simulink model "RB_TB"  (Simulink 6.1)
settings: Solver=ode3  SolverMode=SingleTasking  StartTime=0  StopTime=0.1  FixedStep=0.01  RelTol=1e-3
libraries: simulink x2
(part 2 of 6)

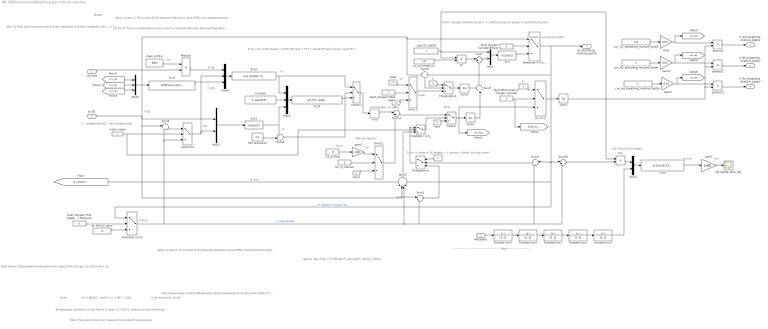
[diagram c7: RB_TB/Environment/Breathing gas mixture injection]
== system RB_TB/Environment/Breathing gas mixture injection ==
  note: Model:
  note: Valve_mode=1; The model of O2 pressure reduction valve (PRV) not compensated to ambient pressure (Drager Dolphin circuit).
  note: K
  note: Flow = Fs, when Pamb < 0.5*P_IM Flow = Fs*(1 -exp(9.5*log(k(i))))/(1 -exp(9.5*log(0.5))) Flow = 0 when P_IM <= P_BL Flow = 0 when P_O2_bottle <= P_IM
  note: Flow
  note: Fs
  note: P_BL
  note: P_breathing_mixture_bottle
  note: Valve_mode=0; The model of O2 pressure reduction valve (PRV) compensated to ambient pressure (Ray circuit).
  note: P_IM_sl
  note: 1 - compensated 0 - not compensated
  note: Fault: "Oxygen Cylinder Empty" = 1 Bottle pressure equals to ambient pressure
  note: l/s
  note: Leaks
  note: Flow = 0 when P_O2_bottle < P_spring + Pamb (for Ray valve)
  note: approx. Ray Flow = Fs*(Pamb+P_spring)/(P_spring + Patm)
  note: pure oxygen, l/s
  note: um
  note: bar
  note: Temperature correction of the flow is (t_amb +273)/273, where t_amb is the temperature of the gas in balloon in deg. C
  note: Note: the system does not measure the ambient temperature
  note: Flow theory: http://www.therebreathersite.nl/gas_flow_through_an_orifice.htm Sonic flow D = d^2*po*A, where d is orifice diameter in mm; p0 = intermediate pressure (input orifice pressure), in bar; A is constant. A = A_O2*cnc_O2+ A_N2*cnc_N2+A_He*cnc_He, where A_O2 = 8.65, A_N2=9.233, A_He=20.71 are constants; cnc_O2, cnc_N2 and cnc_He is concentration of O2, N2 and He ( N2/O2 : He/O2 == 1.067 2.394)
  note: Max O2 flow must be more than the set metabolic rate Max metabolic rate = 0.1 /ls
  note: P_IM
  note: l/s
  note: Life Time of O2 bottele
  note: second
  note: min
  note: ------------------------------------------------- filter------------------------------------------------
  note: Manual injector
  note: l/min
  note: 21_02_07 The uncompensated valve means a Constant Absolute Pressure Regulator. The compensated one is a Constant Ambient Pressure Regulator.
  note: http://www.ckgas.com/html/Rotameters-Basic-Flowmeter-Principles.html Table of Flow Rate Factors For Gases Other Than Air: Gas Factor Air 1 Carbob Dioxide 1.23 Helium 0.37 Nitrogen 0.98 Oxygen 1.05 (N2/O2 : He/O2 == 1. 071 : 2.838) (N2/Air : He/Air == 1. 020 : 2.703)
  note: for ( N2/O2 : He/O2 == 1.067 : 2.83)
  note: A_He should be 24.48
  note: Note:
  note: A_gas
  Orf_size : Inport  Port=1  LatchInput=off
  pr_BL : Inport  Port=2  LatchInput=off
  Metabolic : Inport  Port=3  LatchInput=off
  >=0 : DeadZone  LowerValue=-inf  UpperValue=0
  Fcn : Fcn  Expr=u(2)/u(1)
  Fcn1 : Fcn  Expr=u(1)/u(2)
  Fcn2 : Fcn  Expr=(u(1)/1000)^2*u(2)*u(3)/60
  Fcn3 : Fcn  Expr=8.65*u(1)+9.33*u(2)+24.48*u(3)
  Fcn4 : Fcn  Expr=u(1)/(u(2)+0.0000001)-300
  Fcn5 : Fcn  Expr=u(1)*(1 -exp(9.5*log(u(3))))/u(2)
  Gain : Gain  Gain=0.01
  Gain1 : Gain  Gain=0.01
  Gain2 : Gain  Gain=0.01
  Leak : Constant  Value=2.5
  Mux : Mux  Inputs=2
  Mux1 : Mux  Inputs=2
  Mux2 : Mux  Inputs=3
  Mux3 : Mux  Inputs=2
  Mux4 : Mux  Inputs=3
  Mux5 : Mux  Inputs=3
  O2_bottle_time_life : Scope
  O2_in_flow : Constant  Value=75
  O2_in_manual : Constant  Value=0
  Pr : Product
  Pr1 : Product
  Product : Product
  Sum : Sum  Inputs=|+-
  Sum1 : Sum  Inputs=|-+
  Sum10 : Sum  Inputs=|+-
  Sum11 : Sum  Inputs=|++
  Sum2 : Sum  Orientation=left  Inputs=|-+
  Sum3 : Sum  Inputs=|++
  Sum4 : Sum  Inputs=-+|
  Sum5 : Sum  Orientation=up  Inputs=+--+
  Sum7 : Sum  Orientation=up  Inputs=++|
  Sum8 : Sum  Orientation=down  Inputs=+-
  Switch : Switch  Criteria=u2 > Threshold
  Switch3 : Switch  Criteria=u2 > Threshold
  Threshold=0 : Switch  Orientation=left  Criteria=u2 > Threshold
  Threshold=0_ : Switch  Criteria=u2 > Threshold
  Transfer Fcn{1..5} (5 alike) : TransferFcn  Denominator=[1 1]
  cnc_He_breathing_mixture_bottle : Constant  Value=0
  cnc_N2_breathing_mixture_bottle : Constant  Value=0
  cnc_O2_breathing_mixture_bottle : Constant  Value=100
  constant : Constant  Value=1 -exp(9.5*log(0.5))
  diam_orifice : Constant  Value=400
  fault_Oxygen Cylinder Empty : Constant  Value=0
  fault_Oxygen First Stage Over Pressure : Constant  Value=0
  fault_Oxygen Hose Leaks : Constant  Value=0
  fault_Wrong Gas in Oxygen cylinder : Constant  Value=0
  gain1 : Gain  Gain=1/60
  gain2 : Gain  Gain=1/60
  half pressure1 : Constant  Value=0.5
  pr_IM_O2_valve : Constant  Value=10
  pr_O2_bottle_ini : Constant  Value=230
  product : Product
  product1 : Product
  product2 : Product
  size_O2_bottle : Constant  Value=3
  sum1 : Integrator
  sum2 : Integrator
  sum3 : Integrator
  th = 0.5 : Switch  Criteria=u2 > Threshold  Threshold=0.5
  th=0.5 : Switch  Criteria=u2 > Threshold  Threshold=0.5
  th=0.5_ : Switch  Criteria=u2 > Threshold  Threshold=0.5
  threshold = 0.5 : Switch  Criteria=u2 > Threshold  Threshold=0.5
  threshold = 0.5_ : Switch  Criteria=u2 > Threshold
  threshold = 0.5__ : Switch  Criteria=u2 > Threshold  Threshold=0.5
  tresh=0.5 : Switch  Criteria=u2 > Threshold  Threshold=0.5
  valve_mode : Constant
  z : Constant  Value=0
  z_ : Constant  Value=0
  zero : Constant  Value=0
  zero1 : Constant  Value=0
  zero_ : Constant  Value=0
  zero__ : Constant  Orientation=left  Value=0
  pr_breathing_mixture_bottle : Outport
  V_O2_breathing_mixture_bottle : Outport  Port=2
  V_N2_breathing_mixture_bottle : Outport  Port=3
  V_He_breathing_mixture_bottle : Outport  Port=4
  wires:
  Sum/1 -> Mux/2
  size_O2_bottle/1 -> Mux/1, Pr/1, Pr1/1
  Mux/1 -> Fcn/1
  Pr/1 -> Sum/1
  pr_O2_bottle_ini/1 -> Pr/2
  sum1/1 -> Sum7/2
  pr_BL/1 -> Mux1/1, threshold = 0.5__/1, Sum8/1, Sum5/2, Sum1/1, Sum3/1
  zero/1 -> Switch/3
  Switch3/1 -> >=0/1
  threshold = 0.5/1 -> Sum5/3, Sum1/2, Sum2/2, Sum10/2, Sum3/2, tresh=0.5/3  "pr_intermediate"
  [pr_ambient_sea_level] -> Sum5/1  "pr_atm"
  half pressure1/1 -> Sum4/2
  Mux1/1 -> Fcn1/1
  Mux2/1 -> Fcn5/1
  Sum4/1 -> Switch3/2
  constant/1 -> Mux2/2
  Fcn5/1 -> Switch3/3
  threshold = 0.5__/1 -> Sum8/2, Sum2/1, threshold = 0.5/1, Sum5/4, Sum10/1, pr_breathing_mixture_bottle/1  "pr_breathing_mixture_bottle"
  Fcn/1 -> threshold = 0.5__/3
  fault_Oxygen Cylinder Empty/1 -> threshold = 0.5__/2
  Sum2/1 -> Threshold=0/2
  zero__/1 -> Threshold=0/1
  threshold = 0.5_/1 -> Switch/2
  Sum1/1 -> Threshold=0/3
  Threshold=0/1 -> threshold = 0.5_/1
  Sum5/1 -> threshold = 0.5_/3
  fault_Oxygen First Stage Over Pressure/1 -> threshold = 0.5/2
  fault_Oxygen Hose Leaks/1 -> th=0.5/2
  zero_/1 -> th=0.5/3
  Leak/1 -> th=0.5/1
  Sum7/1 -> Sum/2
  >=0/1 -> Sum11/1
  Sum8/1 -> Threshold=0_/2
  z/1 -> Threshold=0_/1
  th=0.5/1 -> Threshold=0_/3
  sum2/1 -> Sum7/1
  Threshold=0_/1 -> sum2/1
  fault_Wrong Gas in Oxygen cylinder/1 -> th = 0.5/2, [Fault_O2_wrong]
  z_/1 -> th = 0.5/1
  th = 0.5/1 -> sum3/1
  sum3/1 -> product2/2, product1/2, product/2
  Mux4/1 -> Fcn2/1
  valve_mode/1 -> tresh=0.5/2, threshold = 0.5_/2
  Fcn1/1 -> Sum4/1, Mux2/3
  Fcn2/1 -> Mux2/1, Switch3/1
  Product/1 -> Mux4/1
  diam_orifice/1 -> Product/1
  pr_IM_O2_valve/1 -> threshold = 0.5/3
  O2_in_manual/1 -> th=0.5_/2
  zero1/1 -> th=0.5_/3
  Switch/1 -> sum1/1, th = 0.5/3, [O2_flow]
  th=0.5_/1 -> Sum11/2
  Mux3/1 -> Fcn4/1
  Pr1/1 -> Mux3/1
  Metabolic/1 -> Transfer Fcn5/1
  Transfer Fcn2/1 -> Transfer Fcn1/1
  Transfer Fcn1/1 -> Transfer Fcn3/1
  Transfer Fcn5/1 -> Transfer Fcn4/1
  Transfer Fcn4/1 -> Transfer Fcn2/1
  Fcn4/1 -> gain1/1
  gain1/1 -> O2_bottle_time_life/1
  Sum10/1 -> Pr1/2
  Transfer Fcn3/1 -> Mux3/2
  gain2/1 -> th=0.5_/1
  O2_in_flow/1 -> gain2/1
  Sum11/1 -> Switch/1
  Orf_size/1 -> Product/2
  tresh=0.5/1 -> Mux4/2, Mux1/2
  Sum3/1 -> tresh=0.5/1
  Fcn3/1 -> Mux4/3
  Mux5/1 -> Fcn3/1
  cnc_O2_breathing_mixture_bottle/1 -> Gain/1
  Gain/1 -> product/1, [cnc_O2]
  product/1 -> V_O2_breathing_mixture_bottle/1
  cnc_N2_breathing_mixture_bottle/1 -> Gain1/1
  Gain1/1 -> product1/1, [cnc_N2]
  product1/1 -> V_N2_breathing_mixture_bottle/1
  product2/1 -> V_He_breathing_mixture_bottle/1
  cnc_He_breathing_mixture_bottle/1 -> Gain2/1
  Gain2/1 -> product2/1, [cnc_He]
  [cnc_O2] -> Mux5/1
  [cnc_He] -> Mux5/3
  [cnc_N2] -> Mux5/2

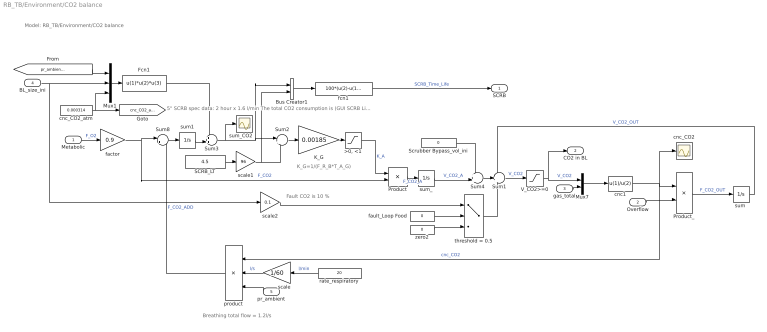
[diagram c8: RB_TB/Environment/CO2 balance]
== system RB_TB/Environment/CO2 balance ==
  note: Model: RB_TB/Environment/CO2 balance
  note: K_G=1/(F_R_B*T_A_G)
  note: Breathing total flow = 1.2l/s
  note: 5" SCRB spec data: 2 hour x 1.6 l/min The total CO2 consumption is (GUI SCRB Life-Time) x 192 / 2 litre
  note: Fault CO2 is 10 %
  Metabolic : Inport  Port=1  LatchInput=off
  Overflow : Inport  Port=2  LatchInput=off
  gas_total : Inport  Port=3  LatchInput=off
  BL_size_ini : Inport  Port=4  LatchInput=off
  pr_ambient : Inport  Orientation=left  Port=5  LatchInput=off
  ">0, <1" : Saturate  UpperLimit=1  LowerLimit=0
  Bus Creator1 : BusCreator  DialogController=Simulink.DDGSource_Bus  Inputs=2
  Fcn1 : Fcn  Expr=u(1)*u(2)*u(3)
  K_G : Gain  Gain=0.00185
  Mux1 : Mux  Inputs=3
  Mux7 : Mux  Inputs=2
  Product : Product
  Product_ : Product
  SCRB_LT : Constant  Value=4.5
  Scrubber Bypass_vol_ini : Constant  Value=0
  Sum1 : Sum  Inputs=-++
  Sum2 : Sum  Inputs=|+-
  Sum3 : Sum  Inputs=++|
  Sum4 : Sum  Inputs=++|
  Sum8 : Sum  Inputs=|++
  V_CO2>=0 : Saturate  UpperLimit=inf  LowerLimit=0
  cnc1 : Fcn  Tag=ee  Priority=306454640  Expr=u(1)/u(2)
  cnc_CO2 : Scope
  cnc_CO2_atm : Constant  Value=0.000314
  factor : Gain  Gain=0.9
  fault_Loop Food : Constant  Value=0
  fcn1 : Fcn  Expr=100*(u(2)-u(1))/u(2)
  product : Product  Orientation=left  Inputs=3
  rate_respiratory : Constant  Orientation=left  Value=20
  scale : Gain  Orientation=left  Gain=1/60
  scale1 : Gain  Gain=96
  scale2 : Gain  Gain=0.1
  "sum " : Integrator
  sum1 : Integrator
  sum_ : Integrator
  sum_CO2 : Scope
  threshold = 0.5 : Switch  Criteria=u2 > Threshold  Threshold=0.5
  zero2 : Constant  Value=0
  SCRB : Outport
  CO2 in BL : Outport  Port=2
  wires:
  Sum2/1 -> K_G/1
  K_G/1 -> ">0, <1"/1
  ">0, <1"/1 -> Product/1  "K_A"
  Product/1 -> sum_/1  "F_CO2_A"
  Sum1/1 -> V_CO2>=0/1  "V_CO2"
  Product_/1 -> "sum "/1  "F_CO2_OUT"
  "sum "/1 -> Sum1/1  "V_CO2_OUT"
  V_CO2>=0/1 -> Mux7/1, CO2 in BL/1  "V_CO2"
  Sum8/1 -> sum1/1
  Sum3/1 -> Sum2/1, Bus Creator1/1, sum_CO2/1
  rate_respiratory/1 -> scale/1  "l/min"
  scale/1 -> product/2  "l/s"
  cnc_CO2_atm/1 -> [cnc_CO2_atm], Mux1/3
  BL_size_ini/1 -> scale2/1, Mux1/2
  SCRB_LT/1 -> scale1/1
  Bus Creator1/1 -> fcn1/1
  fcn1/1 -> SCRB/1  "SCRB_Time_Life"
  scale1/1 -> Sum2/2, Bus Creator1/2
  threshold = 0.5/1 -> Sum1/3
  fault_Loop Food/1 -> threshold = 0.5/2
  scale2/1 -> threshold = 0.5/1
  zero2/1 -> threshold = 0.5/3
  Mux7/1 -> cnc1/1
  cnc1/1 -> cnc_CO2/1, Product_/1, product/1  "cnc_CO2"
  Overflow/1 -> Product_/2
  gas_total/1 -> Mux7/2
  [pr_ambient_sea_level] -> Mux1/1
  Mux1/1 -> Fcn1/1
  product/1 -> Sum8/2  "F_CO2_ADD"
  sum1/1 -> Sum3/2
  Fcn1/1 -> Sum3/1
  Sum4/1 -> Sum1/2
  sum_/1 -> Sum4/2  "V_CO2_A"
  Scrubber Bypass_vol_ini/1 -> Sum4/1
  pr_ambient/1 -> product/3
  factor/1 -> Sum8/1, Product/2  "F_CO2"
  Metabolic/1 -> factor/1  "F_O2"

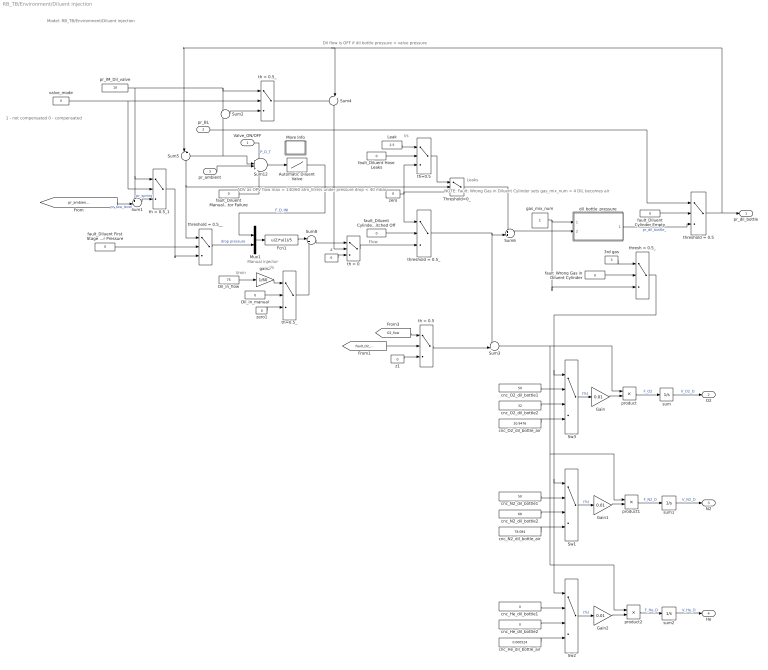
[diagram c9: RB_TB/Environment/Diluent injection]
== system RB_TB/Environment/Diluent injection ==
  note: Model: RB_TB/Environment/Diluent injection
  note: NOTE: Fault: Wrong Gas in Diluent Cylinder sets gas_mix_num = 4 DIL becomes air
  note: Dil flow is OFF if dil bottle pressure < valve pressure
  note: 1 - not compensated 0 - compensated
  note: l/s
  note: Leaks
  note: Flow
  note: l/s
  note: Manual injector
  note: l/min
  note: ADV as OPV flow max = 140/60 atm_litre/s under pressure drop < 40 mbar
  Valve_ON/OFF : Inport  Port=1  LatchInput=off
  pr_BL : Inport  Port=2  LatchInput=off
  pr_ambient : Inport  Port=3  LatchInput=off
  3rd gas : Constant  Value=3
  Automatic Diluent Valve : Lookup  DialogController=Simulink.DDGSource  InputValues=[-1000 0.039 0.04 0.3 1000]  OutputValues=[0 0 70 140 140]/60  LookUpMeth=Interpolation-Use End Values
  Dil_in_flow : Constant  Value=75
  Dil_in_manual : Constant  Value=0
  Fcn1 : Fcn  Expr=u(2)*u(1)/5
  Gain : Gain  Gain=0.01
  Gain1 : Gain  Gain=0.01
  Gain2 : Gain  Gain=0.01
  Leak : Constant  Value=2.5
  More Info : Subsystem
  Mux1 : Mux  Inputs=2
  Sum1 : Sum  Inputs=+-|
  Sum12 : Sum  Inputs=+-++
  Sum2 : Sum
  Sum3 : Sum  Inputs=++|
  Sum4 : Sum  Orientation=down  Inputs=-+|
  Sum5 : Sum  Orientation=down  Inputs=|+-
  Sum6 : Sum  Inputs=++|
  Sum8 : Sum  Inputs=|++
  Sw1 : MultiPortSwitch  Inputs=3
  Sw2 : MultiPortSwitch  Inputs=3
  Sw3 : MultiPortSwitch  Inputs=3
  Threshold=0_ : Switch  Criteria=u2 > Threshold
  cnc_He_dil_bottle1 : Constant  Value=0
  cnc_He_dil_bottle2 : Constant  Value=0
  cnc_He_dil_bottle_air : Constant  Value=0.000524
  cnc_N2_dil_bottle1 : Constant  Value=50
  cnc_N2_dil_bottle2 : Constant  Value=68
  cnc_N2_dil_bottle_air : Constant  Value=78.084
  cnc_O2_dil_bottle1 : Constant  Value=50
  cnc_O2_dil_bottle2 : Constant  Value=32
  cnc_O2_dil_bottle_air : Constant  Value=20.9476
  dil_bottle_pressure : Subsystem
  fault_Diluent Cylinder Empty : Constant  Value=0
  fault_Diluent Cylinder Switched Off : Constant  Value=0
  fault_Diluent First Stage Over Pressure : Constant  Value=0
  fault_Diluent Hose Leaks : Constant  Value=0
  fault_Diluent Manual Injector Failure : Constant  Value=0
  fault_Wrong Gas in Diluent Cylinder : Constant  Value=0
  gain2 : Gain  Gain=1/60
  gas_mix_num : Constant
  pr_IM_Dil_valve : Constant  Value=10
  product : Product
  product1 : Product
  product2 : Product
  sum : Integrator
  sum1 : Integrator
  sum2 : Integrator
  th = 0 : Switch  Criteria=u2 > Threshold
  th = 0.5 : Switch  Criteria=u2 > Threshold  Threshold=0.5
  th = 0.5_ : Switch  Criteria=u2 > Threshold
  th = 0.5_1 : Switch  Criteria=u2 > Threshold
  th=0.5 : Switch  Criteria=u2 > Threshold  Threshold=0.5
  th=0.5_ : Switch  Criteria=u2 > Threshold  Threshold=0.5
  thresh = 0.5_ : Switch  Criteria=u2 > Threshold  Threshold=0.5
  threshold = 0.5 : Switch  Criteria=u2 > Threshold  Threshold=0.5
  threshold = 0.5_ : Switch  Criteria=u2 > Threshold  Threshold=0.5
  threshold = 0.5__ : Switch  Criteria=u2 > Threshold  Threshold=0.5
  valve_mode : Constant  Value=0
  z : Constant  Value=0
  z1 : Constant  Value=0
  zero : Constant  Value=0
  zero1 : Constant  Value=0
  pr_dil_bottle : Outport
  O2 : Outport  Port=2
  N2 : Outport  Port=3
  He : Outport  Port=4
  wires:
  zero/1 -> Threshold=0_/3, th=0.5/3, threshold = 0.5_/1
  gas_mix_num/1 -> dil_bottle_pressure/1(gas_mix), thresh = 0.5_/3
  product/1 -> sum/1  "F_O2"
  sum/1 -> O2/1  "V_O2_D"
  sum1/1 -> N2/1  "V_N2_D"
  product1/1 -> sum1/1  "F_N2_D"
  sum2/1 -> He/1  "V_He_D"
  product2/1 -> sum2/1  "F_He_D"
  cnc_N2_dil_bottle2/1 -> Sw1/3
  cnc_O2_dil_bottle1/1 -> Sw3/2
  Sw3/1 -> Gain/1  "(%)"
  Gain/1 -> product/2
  Gain1/1 -> product1/2
  Gain2/1 -> product2/2
  Sw2/1 -> Gain2/1  "(%)"
  dil_bottle_pressure/1(O2) -> threshold = 0.5/3  "pr_dil_bottle_"
  cnc_O2_dil_bottle2/1 -> Sw3/3
  cnc_N2_dil_bottle1/1 -> Sw1/2
  cnc_He_dil_bottle1/1 -> Sw2/2
  cnc_He_dil_bottle2/1 -> Sw2/3
  threshold = 0.5/1 -> pr_dil_bottle/1, Sum5/1, Sum4/2
  fault_Diluent Cylinder Empty/1 -> threshold = 0.5/2
  z/1 -> th = 0/3
  pr_BL/1 -> Sum12/2, Sum5/2, threshold = 0.5/1, Sum2/2
  fault_Diluent Cylinder Switched Off/1 -> threshold = 0.5_/2
  threshold = 0.5_/1 -> Sum6/2, Sum3/1
  Sw1/1 -> Gain1/1  "(%)"
  cnc_O2_dil_bottle_air/1 -> Sw3/4
  cnc_N2_dil_bottle_air/1 -> Sw1/4
  cnc_He_dil_bottle_air/1 -> Sw2/4
  [O2_flow] -> th = 0.5/1
  [Fault_O2_wrong] -> th = 0.5/2
  z1/1 -> th = 0.5/3
  th = 0.5/1 -> Sum3/2
  Sum3/1 -> product1/1, product2/1, product/1
  valve_mode/1 -> th = 0.5_/2, th = 0.5_1/2
  Sum2/1 -> th = 0.5_/3
  Sum4/1 -> th = 0/2
  Mux1/1 -> Fcn1/1
  fault_Diluent First Stage Over Pressure/1 -> threshold = 0.5__/2
  threshold = 0.5__/1 -> Mux1/2  "drop pressure"
  Sum5/1 -> threshold = 0.5__/1, Threshold=0_/2
  fault_Diluent Hose Leaks/1 -> th=0.5/2
  Leak/1 -> th=0.5/1
  Sum6/1 -> dil_bottle_pressure/2(F_D)
  Threshold=0_/1 -> Sum6/1
  th=0.5/1 -> Threshold=0_/1
  pr_IM_Dil_valve/1 -> th = 0.5_/1, Sum2/1, th = 0.5_1/1, Sum1/1
  th = 0.5_/1 -> Sum4/1
  th = 0.5_1/1 -> threshold = 0.5__/3
  [pr_ambient_sea_level] -> Sum1/2  "pr_sea_level"
  Sum1/1 -> th = 0.5_1/3  "pr_spring"
  fault_Wrong Gas in Diluent Cylinder/1 -> thresh = 0.5_/2
  3rd gas/1 -> thresh = 0.5_/1
  thresh = 0.5_/1 -> Sw3/1, Sw1/1, Sw2/1
  pr_ambient/1 -> Sum12/3
  fault_Diluent Manual Injector Failure/1 -> Sum12/4
  Sum12/1 -> Automatic Diluent Valve/1
  Dil_in_manual/1 -> th=0.5_/2
  zero1/1 -> th=0.5_/3
  th=0.5_/1 -> Sum8/2
  gain2/1 -> th=0.5_/1
  Dil_in_flow/1 -> gain2/1
  Fcn1/1 -> Sum8/1
  Sum8/1 -> th = 0/1
  th = 0/1 -> threshold = 0.5_/3
  Automatic Diluent Valve/1 -> Mux1/1  "F_D_INI"
  Valve_ON/OFF/1 -> Sum12/1  "P_D_T"

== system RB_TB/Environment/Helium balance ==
  note: V_He_BL_ini
  note: Model: RB_TB/Environment/Helium balance
  V_He_breathing : Inport  Port=1  LatchInput=off
  V_He_dil : Inport  Port=2  LatchInput=off
  gas_total : Inport  Port=3  LatchInput=off
  Overflow : Inport  Port=4  LatchInput=off
  BL_size_ini : Inport  Port=5  LatchInput=off
  Fcn1 : Fcn  Expr=u(1)*u(2)*u(3)
  Mux1 : Mux  Inputs=3
  Mux3 : Mux  Inputs=2
  Product_ : Product
  Sum5 : Sum  Inputs=+++-
  V_He>=0 : Saturate  UpperLimit=inf  LowerLimit=0
  cnc3 : Fcn  Tag=ee  Priority=306454640  Expr=u(1)/u(2)
  cnc_He : Scope
  sum : Integrator
  He in BL : Outport
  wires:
  V_He_dil/1 -> Sum5/2  "V_He_D"
  Fcn1/1 -> Sum5/1
  V_He>=0/1 -> He in BL/1, Mux3/1  "V_He"
  Sum5/1 -> V_He>=0/1  "V_He"
  sum/1 -> Sum5/4  "V_He_OUT"
  Product_/1 -> sum/1  "F_He_OUT"
  Mux3/1 -> cnc3/1
  cnc3/1 -> cnc_He/1, Product_/1, [cnc_He_presize]
  gas_total/1 -> Mux3/2
  Overflow/1 -> Product_/2
  BL_size_ini/1 -> Mux1/2
  [pr_ambient_sea_level] -> Mux1/1
  Mux1/1 -> Fcn1/1
  [cnc_He_atm] -> Mux1/3
  V_He_breathing/1 -> Sum5/3

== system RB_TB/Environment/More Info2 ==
  note: Humidity: The water in breathing and from the chemical reaction maintain the humidity constantly at 100%. The situation in open circuit is different, the gas mixture is completely dry, and the diver loses a big quantity of liquids during the dive.

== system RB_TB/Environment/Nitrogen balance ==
  note: Model: RB_TB/Environment/Nitrogen balance
  V_N2_breathing : Inport  Port=1  LatchInput=off
  V_N2_dil : Inport  Port=2  LatchInput=off
  gas_total : Inport  Port=3  LatchInput=off
  Overflow : Inport  Port=4  LatchInput=off
  BL_size_ini : Inport  Port=5  LatchInput=off
  Display2 : Display
  Fcn1 : Fcn  Expr=u(1)*u(2)*u(3)
  Mux1 : Mux  Inputs=3
  Mux8 : Mux  Inputs=2
  Product_ : Product
  Sum5 : Sum  Inputs=+++-
  V_N2>=0 : Saturate  UpperLimit=inf  LowerLimit=0
  cnc2 : Fcn  Tag=ee  Priority=306454640  Expr=u(1)/u(2)
  cnc_N2 : Scope
  sum : Integrator
  N2 in BL : Outport
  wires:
  Product_/1 -> sum/1  "F_N2_OUT"
  sum/1 -> Display2/1, Sum5/4  "V_N2_OUT"
  Sum5/1 -> V_N2>=0/1  "V_N2"
  V_N2>=0/1 -> Mux8/1, N2 in BL/1  "V_N2"
  Fcn1/1 -> Sum5/1
  V_N2_dil/1 -> Sum5/2  "V_N2_D"
  Mux8/1 -> cnc2/1
  cnc2/1 -> Product_/1, cnc_N2/1, [cnc_N2_presize]
  gas_total/1 -> Mux8/2
  Overflow/1 -> Product_/2
  BL_size_ini/1 -> Mux1/2
  [pr_ambient_sea_level] -> Mux1/1
  Mux1/1 -> Fcn1/1
  [cnc_N2_atm] -> Mux1/3
  V_N2_breathing/1 -> Sum5/3

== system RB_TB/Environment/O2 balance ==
  note: Model: RB_TB/Environment/O2 balance
  V_O2_breathing : Inport  Port=1  LatchInput=off
  V_O2_dil : Inport  Port=2  LatchInput=off
  Metabolic : Inport  Port=3  LatchInput=off
  gas_total : Inport  Port=4  LatchInput=off
  Overflow : Inport  Port=5  LatchInput=off
  BL_size_ini : Inport  Port=6  LatchInput=off
  Fcn1 : Fcn  Expr=u(1)*u(2)*u(3)
  Mux1 : Mux  Inputs=3
  Mux6 : Mux  Inputs=2
  Product : Product
  Sum2 : Sum  Inputs=-+++-
  V_O2>=0 : Saturate  UpperLimit=inf  LowerLimit=0
  cnc : Fcn  Tag=ee  Priority=306454640  Expr=u(1)/u(2)
  cnc_O2 : Scope
  cnc_O2_atm : Constant  Value=0.20948
  sum : Integrator
  sum2 : Integrator
  O2 in BL : Outport
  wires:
  Fcn1/1 -> Sum2/3  "V_O2_ini"
  Product/1 -> sum/1  "F_O2_OUT"
  sum/1 -> Sum2/1  "V_O2_OUT"
  Sum2/1 -> V_O2>=0/1  "V_O2"
  V_O2_breathing/1 -> Sum2/2  "V_O2_O"
  sum2/1 -> Sum2/5  "V_R_B"
  V_O2_dil/1 -> Sum2/4  "V_O2_D"
  Metabolic/1 -> sum2/1  "F_R_B"
  V_O2>=0/1 -> Mux6/1, O2 in BL/1  "V_O2"
  BL_size_ini/1 -> Mux1/2
  cnc_O2_atm/1 -> [cnc_O2_atm], Mux1/3
  Mux6/1 -> cnc/1
  gas_total/1 -> Mux6/2
  cnc/1 -> Product/1, cnc_O2/1
  Overflow/1 -> Product/2
  [pr_ambient_sea_level] -> Mux1/1
  Mux1/1 -> Fcn1/1

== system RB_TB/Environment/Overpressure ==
  note: Model: RB_TB/Environment/Overpressure
  note: OPV flow max = 300/60 (atm_litre)/s under pressure drop < 40 mbar
  Depth : Inport  Port=1  LatchInput=off
  pr_BL : Inport  Port=2  LatchInput=off
  More Info2 : Subsystem
  OverPressure Valve : Lookup  DialogController=Simulink.DDGSource  InputValues=[-1000 0.025 0.04 0.3 1000]  OutputValues=[0 0 300 600 600]/60  LookUpMeth=Interpolation-Use End Values
  Sum12 : Sum  Inputs=|-+
  Sum4 : Sum  Inputs=++|
  x 0.2 : Gain  Gain=0.1
  Overflow : Outport
  pr_ambient : Outport  Port=2
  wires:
  Depth/1 -> x 0.2/1
  Sum4/1 -> Sum12/1, pr_ambient/1
  x 0.2/1 -> Sum4/2  "water pressure"
  Sum12/1 -> OverPressure Valve/1
  [pr_ambient_sea_level] -> Sum4/1  "bar"
  pr_BL/1 -> Sum12/2  "Breathing loop pressure"
  OverPressure Valve/1 -> Overflow/1

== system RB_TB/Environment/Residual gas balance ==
  note: Model: RB_TB/Environment/Residual gas balance gas balance
  note: vol_reminder_BL_ini
  gas_total : Inport  Port=1  LatchInput=off
  Overflow : Inport  Port=2  LatchInput=off
  BL_size_ini : Inport  Port=3  LatchInput=off
  Fcn1 : Fcn  Expr=u(1)*u(2)*u(3)
  Mux1 : Mux  Inputs=3
  Mux9 : Mux  Inputs=2
  Product_ : Product
  Sum5 : Sum  Inputs=|+-
  V_Re>=0 : Saturate  UpperLimit=inf  LowerLimit=0
  cnc4 : Fcn  Tag=ee  Priority=306454640  Expr=u(1)/u(2)
  cnc_res : Scope
  cnc_res_atm : Constant  Value=0.009365
  sum : Integrator
  Re in BL : Outport
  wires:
  sum/1 -> Sum5/2  "V_Re_OUT"
  Sum5/1 -> V_Re>=0/1  "V_Re"
  V_Re>=0/1 -> Re in BL/1, Mux9/1  "V_Re"
  Fcn1/1 -> Sum5/1
  cnc4/1 -> cnc_res/1, Product_/1  "cnc_res"
  Mux9/1 -> cnc4/1
  Product_/1 -> sum/1  "F_Re_OUT"
  Overflow/1 -> Product_/2  "P_OVER"
  gas_total/1 -> Mux9/2
  BL_size_ini/1 -> Mux1/2
  [pr_ambient_sea_level] -> Mux1/1
  Mux1/1 -> Fcn1/1
  cnc_res_atm/1 -> Mux1/3

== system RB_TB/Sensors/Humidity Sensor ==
  note: Model: RB_TB/Sensors/Humidity_sensor
  note: Voltage supply 0-5V
  note: sensor' tau = 1/gain
  note: This subsystem models a digital 5V humidity sensor including 16-bit ADC.
  in : Inport  Port=1  LatchInput=off
  ADC : Subsystem
  Constant : Constant  Value=0.23
  Integrator : Integrator
  Sum2 : Sum  Inputs=++|
  Sum6 : Sum  Inputs=|+-
  TC : Gain  Gain=1/15
  VS : Gain  Gain=5
  out : Outport
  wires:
  TC/1 -> Integrator/1
  Integrator/1 -> Sum2/2
  Constant/1 -> Sum2/1
  Sum2/1 -> VS/1, Sum6/2
  VS/1 -> ADC/1(voltage)
  in/1 -> Sum6/1
  Sum6/1 -> TC/1
  ADC/1(pcm) -> out/1

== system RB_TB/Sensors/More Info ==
  note: one CO2 24(29) bits ~2ms (ADC) for each: -Channel1 -Channel2 -CO2 temerature one He 8bits? PWM two pressure 3.3V 15 Bits 35ms conversion time ~3ms serial interface 16 Temper Stick 5V 24(29) bits ~20ms (ADC) for 16 sensors one Temperature 5V 24(29) bits ~2ms (ADC) one Humidity 5V 24(29) bits Response Time, 1/e-15s ~2ms (ADC) four PPO2 24(29) 6s ~2ms (ADC)
  note: Temporary actions: 1)
  note: This sub system modes the sensors of the Re-Breather Test Bench

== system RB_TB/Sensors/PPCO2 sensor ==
  note: CO2
  note: This subsystem models a digital 5V CO2 sensor including 16-bit ADC.
  note: sensor' tau = 1/gain
  note: Voltage supply 0-5V
  note: Model: RB_TB/Sensors/PPCO2 sensor
  note: 5s time constant
  PPCO2 : Inport  Port=1  LatchInput=off
  ADC : Subsystem
  Integrator : Integrator
  Product : Product
  Sum2 : Sum  Inputs=++|
  Sum6 : Sum  Inputs=|+-
  TC_CO2_REC : Gain  Gain=1/5
  VS_CO2 : Gain  Gain=5
  PPCO2_S : Outport
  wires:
  ADC/1(pcm) -> PPCO2_S/1  "CO2_S"
  Sum6/1 -> TC_CO2_REC/1
  PPCO2/1 -> Sum6/1
  VS_CO2/1 -> ADC/1(voltage)
  Sum2/1 -> VS_CO2/1, Sum6/2
  [cnc_CO2_atm] -> Product/1
  [pr_ambient_sea_level] -> Product/2
  Product/1 -> Sum2/1
  Integrator/1 -> Sum2/2
  TC_CO2_REC/1 -> Integrator/1

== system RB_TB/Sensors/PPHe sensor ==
  note: sensor' tau = 1/gain
  note: Model: RB_TB/Sensors/PPHe sensor
  note: range is 5V/100%
  note: Time constant is 10 s
  note: PPHe
  PPHe : Inport  Port=1  LatchInput=off
  ADC : Subsystem
  Integrator : Integrator
  Mux2 : Mux  Inputs=2
  Product : Product
  Sum : Sum  Inputs=++|
  Sum6 : Sum  Inputs=|+-
  TC_PPHe : Gain  Gain=1/10
  VS_PPHe : Gain  Gain=5
  cnc : Fcn  Tag=ee  Priority=306454640  Expr=u(1)/u(2)
  PPHe_S : Outport
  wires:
  Sum/1 -> Sum6/2, Mux2/1
  Integrator/1 -> Sum/2
  Product/1 -> Sum/1  "PPO2_atm_ini"
  [pr_ambient_sea_level] -> Product/2
  [cnc_He_atm] -> Product/1
  ADC/1(pcm) -> PPHe_S/1
  VS_PPHe/1 -> ADC/1(voltage)  "PPO2_S"
  PPHe/1 -> Sum6/1
  Sum6/1 -> TC_PPHe/1
  TC_PPHe/1 -> Integrator/1
  Mux2/1 -> cnc/1
  [scale_pressure] -> Mux2/2
  cnc/1 -> VS_PPHe/1

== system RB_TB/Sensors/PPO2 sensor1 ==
  note: sensor' tau = 1/gain
  note: Model: RB_TB/Sensors/PPO2 sensor1
  note: Voltage supply = 5V scale = 5V/2.3
  note: Delay 0.1s is removed
  note: PPO2
  note: Time constant is time of 90% / 2.305
  PPO2 : Inport  Port=1  LatchInput=off
  ADC : Subsystem
  Integrator : Integrator
  More Info1 : Subsystem
  Product : Product
  Sum : Sum  Inputs=++|
  Sum6 : Sum  Inputs=|+-
  TS_PPO2_REC : Gain  Gain=1/1.5
  VS_PPO2 : Gain  Gain=5/2.3
  PPO2_S : Outport
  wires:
  Sum/1 -> Sum6/2, VS_PPO2/1
  Integrator/1 -> Sum/2
  Product/1 -> Sum/1  "PPO2_atm_ini"
  [pr_ambient_sea_level] -> Product/2
  [cnc_O2_atm] -> Product/1
  ADC/1(pcm) -> PPO2_S/1
  VS_PPO2/1 -> ADC/1(voltage)  "PPO2_S"
  PPO2/1 -> Sum6/1
  Sum6/1 -> TS_PPO2_REC/1
  TS_PPO2_REC/1 -> Integrator/1

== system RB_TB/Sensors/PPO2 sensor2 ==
  note: PPO2
  note: Delay 0.1s is removed
  note: Voltage supply = 5V scale = 5V/2.3
  note: Model: RB_TB/Sensors/PPO2 sensor2
  note: sensor' tau = 1/gain
  note: Time constant is time of 90% / 2.305
  PPO2 : Inport  Port=1  LatchInput=off
  ADC : Subsystem
  Integrator : Integrator
  More Info1 : Subsystem
  Product : Product
  Sum : Sum  Inputs=++|
  Sum6 : Sum  Inputs=|+-
  TS_PPO2_REC : Gain  Gain=1/1.75
  VS_PPO2 : Gain  Gain=5/2.3
  PPO2_S : Outport
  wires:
  TS_PPO2_REC/1 -> Integrator/1
  Sum6/1 -> TS_PPO2_REC/1
  PPO2/1 -> Sum6/1
  VS_PPO2/1 -> ADC/1(voltage)  "PPO2_S"
  ADC/1(pcm) -> PPO2_S/1
  [cnc_O2_atm] -> Product/1
  [pr_ambient_sea_level] -> Product/2
  Product/1 -> Sum/1  "PPO2_atm_ini"
  Integrator/1 -> Sum/2
  Sum/1 -> VS_PPO2/1, Sum6/2

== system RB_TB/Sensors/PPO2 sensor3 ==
  note: sensor' tau = 1/gain
  note: Model: RB_TB/Sensors/PPO2 sensor3
  note: Voltage supply = 5V scale = 5V/2.3
  note: Delay 0.1s is removed
  note: PPO2
  note: Time constant is time of 90% / 2.305
  PPO2 : Inport  Port=1  LatchInput=off
  ADC : Subsystem
  Integrator : Integrator
  More Info1 : Subsystem
  Product : Product
  Sum : Sum  Inputs=++|
  Sum6 : Sum  Inputs=|+-
  TS_PPO2_REC : Gain  Gain=1/2
  VS_PPO2 : Gain  Gain=5/2.3
  PPO2_S : Outport
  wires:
  Sum/1 -> Sum6/2, VS_PPO2/1
  Integrator/1 -> Sum/2
  Product/1 -> Sum/1  "PPO2_atm_ini"
  [pr_ambient_sea_level] -> Product/2
  [cnc_O2_atm] -> Product/1
  ADC/1(pcm) -> PPO2_S/1
  VS_PPO2/1 -> ADC/1(voltage)  "PPO2_S"
  PPO2/1 -> Sum6/1
  Sum6/1 -> TS_PPO2_REC/1
  TS_PPO2_REC/1 -> Integrator/1

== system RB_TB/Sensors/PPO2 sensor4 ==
  note: PPO2
  note: Delay 0.1s is removed
  note: Voltage supply = 5V scale = 5V/2.3
  note: Model: RB_TB/Sensors/PPO2 sensor4
  note: sensor' tau = 1/gain
  note: Time constant is time of 90% / 2.305
  PPO2 : Inport  Port=1  LatchInput=off
  ADC : Subsystem
  Integrator : Integrator
  More Info1 : Subsystem
  Product : Product
  Sum : Sum  Inputs=++|
  Sum6 : Sum  Inputs=|+-
  TS_PPO2_REC : Gain  Gain=1/2.5
  VS_PPO2 : Gain  Gain=5/2.3
  PPO2_S : Outport
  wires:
  TS_PPO2_REC/1 -> Integrator/1
  Sum6/1 -> TS_PPO2_REC/1
  PPO2/1 -> Sum6/1
  VS_PPO2/1 -> ADC/1(voltage)  "PPO2_S"
  ADC/1(pcm) -> PPO2_S/1
  [cnc_O2_atm] -> Product/1
  [pr_ambient_sea_level] -> Product/2
  Product/1 -> Sum/1  "PPO2_atm_ini"
  Integrator/1 -> Sum/2
  Sum/1 -> VS_PPO2/1, Sum6/2

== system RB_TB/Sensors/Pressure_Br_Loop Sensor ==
  note: 35 ms conversion time
  note: This subsystem models a digital 3V pressure sensor including 15-bit ADC.
  note: Voltage supply 0-5V
  note: Model: RB_TB/Sensors/Pressure_Br_Loop Sensor
  in : Inport  Port=1  LatchInput=off
  ADC : Subsystem
  Mux2 : Mux  Inputs=2
  Transport Delay : TransportDelay  DelayTime=0.035  InitialInput=1.01
  VS : Gain  Gain=3
  cnc : Fcn  Tag=ee  Priority=306454640  Expr=u(1)/u(2)
  out : Outport
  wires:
  Mux2/1 -> cnc/1
  Transport Delay/1 -> Mux2/1
  [scale_pressure] -> Mux2/2
  cnc/1 -> VS/1
  ADC/1(pcm) -> out/1
  VS/1 -> ADC/1(voltage)
  in/1 -> Transport Delay/1  "pressure"

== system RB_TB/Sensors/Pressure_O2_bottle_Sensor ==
  note: Model: RB_TB/Sensors/Pressure_O2_bottle_Sensor
  note: Voltage supply 0-5V
  note: This subsystem models a digital 3V pressure sensor including 15-bit ADC.
  note: 35 ms conversion time
  in : Inport  Port=1  LatchInput=off
  300barRange : Constant  Value=300
  ADC : Subsystem
  Mux2 : Mux  Inputs=2
  Transport Delay : TransportDelay  DelayTime=0.035  InitialInput=1.01
  VS : Gain  Gain=3
  cnc : Fcn  Tag=ee  Priority=306454640  Expr=u(1)/(u(2)+0.000001)
  out : Outport
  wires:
  in/1 -> Transport Delay/1  "pressure"
  VS/1 -> ADC/1(voltage)
  ADC/1(pcm) -> out/1
  cnc/1 -> VS/1
  Transport Delay/1 -> Mux2/1
  Mux2/1 -> cnc/1
  300barRange/1 -> Mux2/2

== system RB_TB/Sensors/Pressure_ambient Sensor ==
  note: Model: RB_TB/Sensors/Pressure_ambient Sensor
  note: Voltage supply 0-5V
  note: This subsystem models a digital 3V pressure sensor including 15-bit ADC.
  note: 35 ms conversion time
  in : Inport  Port=1  LatchInput=off
  ADC : Subsystem
  Mux1 : Mux  Inputs=2
  Mux2 : Mux  Inputs=2
  Transport Delay : TransportDelay  DelayTime=0.035  InitialInput=1.01
  VS : Gain  Gain=3
  cnc : Fcn  Tag=ee  Priority=306454640  Expr=u(1)/u(2)
  cnc1 : Fcn  Tag=ee  Priority=306454640  Expr=u(1)+u(2)/10
  depth_range : Constant  Value=600
  out : Outport
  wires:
  in/1 -> Transport Delay/1  "pressure"
  VS/1 -> ADC/1(voltage)
  ADC/1(pcm) -> out/1
  [pr_ambient_sea_level] -> Mux1/1
  depth_range/1 -> Mux1/2
  cnc/1 -> VS/1
  Mux1/1 -> cnc1/1
  cnc1/1 -> Mux2/2, [scale_pressure]
  Transport Delay/1 -> Mux2/1
  Mux2/1 -> cnc/1

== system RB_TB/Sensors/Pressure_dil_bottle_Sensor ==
  note: 35 ms conversion time
  note: This subsystem models a digital 3V pressure sensor including 15-bit ADC.
  note: Voltage supply 0-5V
  note: Model: RB_TB/Sensors/Pressure_dil_bottle_Sensor
  in : Inport  Port=1  LatchInput=off
  300barRange : Constant  Value=300
  ADC : Subsystem
  Mux2 : Mux  Inputs=2
  Transport Delay : TransportDelay  DelayTime=0.035  InitialInput=1.01
  VS : Gain  Gain=3
  cnc : Fcn  Tag=ee  Priority=306454640  Expr=u(1)/(u(2)+0.000001)
  out : Outport
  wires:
  Mux2/1 -> cnc/1
  Transport Delay/1 -> Mux2/1
  cnc/1 -> VS/1
  ADC/1(pcm) -> out/1
  VS/1 -> ADC/1(voltage)
  in/1 -> Transport Delay/1  "pressure"
  300barRange/1 -> Mux2/2

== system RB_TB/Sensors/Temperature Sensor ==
  note: This subsystem models a digital 5V temperature sensor including 16-bit ADC.
  note: sensor' tau = 1/gain
  note: Voltage supply 0-5V
  note: Model: RB_TB/Sensors/temperature_sensor
  note: deg
  note: V/deg
  in : Inport  Port=1  LatchInput=off
  ADC : Subsystem
  Integrator : Integrator
  Sum2 : Sum  Inputs=++|
  Sum6 : Sum  Inputs=|+-
  TS : Gain  Gain=1/35
  VS : Gain  Gain=5
  sensitivity : Gain  Gain=0.01
  out : Outport
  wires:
  ADC/1(pcm) -> out/1
  Sum6/1 -> TS/1
  VS/1 -> ADC/1(voltage)
  Sum2/1 -> Sum6/2, sensitivity/1
  [temperature_sea_level] -> Sum2/1
  Integrator/1 -> Sum2/2
  TS/1 -> Integrator/1
  sensitivity/1 -> VS/1
  in/1 -> Sum6/1

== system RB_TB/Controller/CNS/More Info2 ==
  note: The NOAA limits for CNS oxygen toxicity are taken from www.dmscuba.com/Oxygen_Toxicity_Calculations.pdf , "Oxygen Toxicity Calculations" by Erik C. Baker, P.E.
  note: ..."The common method in use to "track" CNS oxygen toxicity is to compute a "CNS fraction" for each segment of the dive profile and then sum up these results to produce a total CNS fraction for the dive. These fractions are often multiplied by 100 and expressed as a percentage (CNS %). A CNS fraction is calculated by taking the time spent at a given PO2 and dividing by the NOAA time limit for that PO2. When the CNS fractions from all segments of the dive profile add up to 1 (or 100%) then the overall limit for CNS oxygen toxicity has been reached for that dive. " ..."The problem is that, to my knowledge, a reliable method has not yet been developed to calculate the rate of recovery from oxygen exposure during these periods of intermittent oxygen breathing. This is an area for future research by the academicians. It is, however, a common practice in technical diving to calculate a decay in the CNS fraction during surface intervals using an exponential decay equation with a half-time of 90 minutes.
  note: "Sensor fusion by using a sliding observer for an underwater breathing system" by Salvatore Carotenuto, Luigi Iannelli, Sabato Manfredi, Stefania Santini
  note: ..."(ii) breathing oxygen at high partial pressure (greater than 0.5 [atm]) can be toxic [2] (Central Nervous System (CNS) oxygen toxicity is related to both oxygen pressure level and duration of the exposure [3])."
  note: "Deep Life Ltd"
  note: ..."In conservative mode we add 0.3 and in aggressive mode 0.2, to the actual PPO2 for the purposes of CNS calculation. When the resulting CNS gets to 90%, the model tell the user the system is "Adding an air break" and stop injecting O2 until the PPO2 is breathed down to 0.4, where we maintain a 0.4 setpoint. Then when CNS falls down to 85%, th system return the actual PPO2 to the desired PPO2 set point."

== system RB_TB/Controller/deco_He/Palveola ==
  note: Model: RB_TB/Controller/deco_He/Palveola
  Gas concentration : Inport  Port=1  LatchInput=off
  "depth, m " : Inport  Port=2  LatchInput=off
  Humidity : Inport  Port=3  LatchInput=off
  Temperature : Inport  Port=4  LatchInput=off
  Fcn2 : Fcn  Expr=0
  Mux1 : Mux  Inputs=2
  Product1 : Product
  Sum2 : Sum  Inputs=++|
  Sum5 : Sum  Inputs=++|
  cnc_He_atm : Constant  Value=5.24e-006
  gain1 : Gain  Gain=0.1
  Psw : Outport
  Palv : Outport  Port=2
  P_alv_INI : Outport  Port=3
  fnc_hum_temp : Outport  Port=4
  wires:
  Sum2/1 -> Palv/1  "Alveolar partial pressure of  the gas in the breathing mix"
  Sum5/1 -> Product1/2
  Fcn2/1 -> fnc_hum_temp/1, Sum5/2  "fnc_hum_temp"
  cnc_He_atm/1 -> Sum2/2, P_alv_INI/1, [cnc_He_atm]
  Temperature/1 -> Mux1/2
  Humidity/1 -> Mux1/1
  Mux1/1 -> Fcn2/1
  gain1/1 -> Psw/1, Sum5/1  "pressure of sea water"
  Gas concentration/1 -> Product1/1
  Product1/1 -> Sum2/1
  "depth, m "/1 -> gain1/1

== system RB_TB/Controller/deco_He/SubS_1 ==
  note: Model: RB_TB/Controller/deco_He/SubS_2
  Palv : Inport  Port=1  LatchInput=off
  Pamb_sea : Inport  Port=2  LatchInput=off
  Palv_INI : Inport  Port=3  LatchInput=off
  HT : Inport  Port=4  LatchInput=off
  BC1 : BusCreator  DialogController=Simulink.DDGSource_Bus
  He_a : Constant  Value=1.7443
  He_b : Constant  Value=0.4245
  Mux6 : Mux  Inputs=3
  Product1 : Product
  Sum2 : Sum  Inputs=|+-
  Sum3 : Sum  Inputs=++|
  fcn1 : Fcn  Expr=log(2)/u(1)
  fcn3 : Fcn  Expr=u(3)+u(2)/u(1)
  pr_PHe : TransferFcn  Numerator=[1/60]  Denominator=[1 0]
  bus : Outport
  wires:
  BC1/1 -> bus/1
  pr_PHe/1 -> Sum3/2
  Palv_INI/1 -> Sum3/1
  Sum3/1 -> BC1/2, Sum2/2  "Pt"
  He_a/1 -> Mux6/3  "He_a"
  Pamb_sea/1 -> Mux6/2
  Palv/1 -> Sum2/1
  fcn1/1 -> Product1/1, BC1/1  "He_k"
  Mux6/1 -> fcn3/1
  He_b/1 -> Mux6/1, BC1/3  "He_b"
  fcn3/1 -> BC1/4  "M0"
  Product1/1 -> pr_PHe/1
  Sum2/1 -> Product1/2
  HT/1 -> fcn1/1

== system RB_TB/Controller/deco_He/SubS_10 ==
  note: Model: RB_TB/Controller/deco_He/SubS_2
  Palv : Inport  Port=1  LatchInput=off
  Pamb_sea : Inport  Port=2  LatchInput=off
  Palv_INI : Inport  Port=3  LatchInput=off
  HT : Inport  Port=4  LatchInput=off
  BC1 : BusCreator  DialogController=Simulink.DDGSource_Bus
  He_a : Constant  Value=0.5568
  He_b : Constant  Value=0.8903
  Mux6 : Mux  Inputs=3
  Product1 : Product
  Sum2 : Sum  Inputs=|+-
  Sum3 : Sum  Inputs=++|
  fcn1 : Fcn  Expr=log(2)/u(1)
  fcn3 : Fcn  Expr=u(3)+u(2)/u(1)
  pr_PHe : TransferFcn  Numerator=[1/60]  Denominator=[1 0]
  bus : Outport
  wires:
  HT/1 -> fcn1/1
  Sum2/1 -> Product1/2
  Product1/1 -> pr_PHe/1
  fcn3/1 -> BC1/4  "M0"
  He_b/1 -> BC1/3, Mux6/1  "He_b"
  Mux6/1 -> fcn3/1
  fcn1/1 -> BC1/1, Product1/1  "He_k"
  Palv/1 -> Sum2/1
  Pamb_sea/1 -> Mux6/2
  He_a/1 -> Mux6/3  "He_a"
  Sum3/1 -> Sum2/2, BC1/2  "Pt"
  Palv_INI/1 -> Sum3/1
  pr_PHe/1 -> Sum3/2
  BC1/1 -> bus/1

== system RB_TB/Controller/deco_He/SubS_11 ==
  note: Model: RB_TB/Controller/deco_He/SubS_2
  Palv : Inport  Port=1  LatchInput=off
  Pamb_sea : Inport  Port=2  LatchInput=off
  Palv_INI : Inport  Port=3  LatchInput=off
  HT : Inport  Port=4  LatchInput=off
  BC1 : BusCreator  DialogController=Simulink.DDGSource_Bus
  He_a : Constant  Value=0.5285
  He_b : Constant  Value=0.8997
  Mux6 : Mux  Inputs=3
  Product1 : Product
  Sum2 : Sum  Inputs=|+-
  Sum3 : Sum  Inputs=++|
  fcn1 : Fcn  Expr=log(2)/u(1)
  fcn3 : Fcn  Expr=u(3)+u(2)/u(1)
  pr_PHe : TransferFcn  Numerator=[1/60]  Denominator=[1 0]
  bus : Outport
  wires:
  BC1/1 -> bus/1
  pr_PHe/1 -> Sum3/2
  Palv_INI/1 -> Sum3/1
  Sum3/1 -> BC1/2, Sum2/2  "Pt"
  He_a/1 -> Mux6/3  "He_a"
  Pamb_sea/1 -> Mux6/2
  Palv/1 -> Sum2/1
  fcn1/1 -> Product1/1, BC1/1  "He_k"
  Mux6/1 -> fcn3/1
  He_b/1 -> Mux6/1, BC1/3  "He_b"
  fcn3/1 -> BC1/4  "M0"
  Product1/1 -> pr_PHe/1
  Sum2/1 -> Product1/2
  HT/1 -> fcn1/1

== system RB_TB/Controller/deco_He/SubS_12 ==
  note: Model: RB_TB/Controller/deco_He/SubS_2
  Palv : Inport  Port=1  LatchInput=off
  Pamb_sea : Inport  Port=2  LatchInput=off
  Palv_INI : Inport  Port=3  LatchInput=off
  HT : Inport  Port=4  LatchInput=off
  BC1 : BusCreator  DialogController=Simulink.DDGSource_Bus
  He_a : Constant  Value=0.5178
  He_b : Constant  Value=0.9073
  Mux6 : Mux  Inputs=3
  Product1 : Product
  Sum2 : Sum  Inputs=|+-
  Sum3 : Sum  Inputs=++|
  fcn1 : Fcn  Expr=log(2)/u(1)
  fcn3 : Fcn  Expr=u(3)+u(2)/u(1)
  pr_PHe : TransferFcn  Numerator=[1/60]  Denominator=[1 0]
  bus : Outport
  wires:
  HT/1 -> fcn1/1
  Sum2/1 -> Product1/2
  Product1/1 -> pr_PHe/1
  fcn3/1 -> BC1/4  "M0"
  He_b/1 -> BC1/3, Mux6/1  "He_b"
  Mux6/1 -> fcn3/1
  fcn1/1 -> BC1/1, Product1/1  "He_k"
  Palv/1 -> Sum2/1
  Pamb_sea/1 -> Mux6/2
  He_a/1 -> Mux6/3  "He_a"
  Sum3/1 -> Sum2/2, BC1/2  "Pt"
  Palv_INI/1 -> Sum3/1
  pr_PHe/1 -> Sum3/2
  BC1/1 -> bus/1

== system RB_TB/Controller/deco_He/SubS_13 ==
  note: Model: RB_TB/Controller/deco_He/SubS_2
  Palv : Inport  Port=1  LatchInput=off
  Pamb_sea : Inport  Port=2  LatchInput=off
  Palv_INI : Inport  Port=3  LatchInput=off
  HT : Inport  Port=4  LatchInput=off
  BC1 : BusCreator  DialogController=Simulink.DDGSource_Bus
  He_a : Constant  Value=0.5137
  He_b : Constant  Value=0.9122
  Mux6 : Mux  Inputs=3
  Product1 : Product
  Sum2 : Sum  Inputs=|+-
  Sum3 : Sum  Inputs=++|
  fcn1 : Fcn  Expr=log(2)/u(1)
  fcn3 : Fcn  Expr=u(3)+u(2)/u(1)
  pr_PHe : TransferFcn  Numerator=[1/60]  Denominator=[1 0]
  bus : Outport
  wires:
  BC1/1 -> bus/1
  pr_PHe/1 -> Sum3/2
  Palv_INI/1 -> Sum3/1
  Sum3/1 -> BC1/2, Sum2/2  "Pt"
  He_a/1 -> Mux6/3  "He_a"
  Pamb_sea/1 -> Mux6/2
  Palv/1 -> Sum2/1
  fcn1/1 -> Product1/1, BC1/1  "He_k"
  Mux6/1 -> fcn3/1
  He_b/1 -> Mux6/1, BC1/3  "He_b"
  fcn3/1 -> BC1/4  "M0"
  Product1/1 -> pr_PHe/1
  Sum2/1 -> Product1/2
  HT/1 -> fcn1/1

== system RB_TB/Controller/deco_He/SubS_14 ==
  note: Model: RB_TB/Controller/deco_He/SubS_2
  Palv : Inport  Port=1  LatchInput=off
  Pamb_sea : Inport  Port=2  LatchInput=off
  Palv_INI : Inport  Port=3  LatchInput=off
  HT : Inport  Port=4  LatchInput=off
  BC1 : BusCreator  DialogController=Simulink.DDGSource_Bus
  He_a : Constant  Value=0.5196
  He_b : Constant  Value=0.9171
  Mux6 : Mux  Inputs=3
  Product1 : Product
  Sum2 : Sum  Inputs=|+-
  Sum3 : Sum  Inputs=++|
  fcn1 : Fcn  Expr=log(2)/u(1)
  fcn3 : Fcn  Expr=u(3)+u(2)/u(1)
  pr_PHe : TransferFcn  Numerator=[1/60]  Denominator=[1 0]
  bus : Outport
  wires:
  HT/1 -> fcn1/1
  Sum2/1 -> Product1/2
  Product1/1 -> pr_PHe/1
  fcn3/1 -> BC1/4  "M0"
  He_b/1 -> BC1/3, Mux6/1  "He_b"
  Mux6/1 -> fcn3/1
  fcn1/1 -> BC1/1, Product1/1  "He_k"
  Palv/1 -> Sum2/1
  Pamb_sea/1 -> Mux6/2
  He_a/1 -> Mux6/3  "He_a"
  Sum3/1 -> Sum2/2, BC1/2  "Pt"
  Palv_INI/1 -> Sum3/1
  pr_PHe/1 -> Sum3/2
  BC1/1 -> bus/1

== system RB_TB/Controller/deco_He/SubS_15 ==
  note: Model: RB_TB/Controller/deco_He/SubS_2
  Palv : Inport  Port=1  LatchInput=off
  Pamb_sea : Inport  Port=2  LatchInput=off
  Palv_INI : Inport  Port=3  LatchInput=off
  HT : Inport  Port=4  LatchInput=off
  BC1 : BusCreator  DialogController=Simulink.DDGSource_Bus
  He_a : Constant  Value=0.515
  He_b : Constant  Value=0.9217
  Mux6 : Mux  Inputs=3
  Product1 : Product
  Sum2 : Sum  Inputs=|+-
  Sum3 : Sum  Inputs=++|
  fcn1 : Fcn  Expr=log(2)/u(1)
  fcn3 : Fcn  Expr=u(3)+u(2)/u(1)
  pr_PHe : TransferFcn  Numerator=[1/60]  Denominator=[1 0]
  bus : Outport
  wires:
  BC1/1 -> bus/1
  pr_PHe/1 -> Sum3/2
  Palv_INI/1 -> Sum3/1
  Sum3/1 -> BC1/2, Sum2/2  "Pt"
  He_a/1 -> Mux6/3  "He_a"
  Pamb_sea/1 -> Mux6/2
  Palv/1 -> Sum2/1
  fcn1/1 -> Product1/1, BC1/1  "He_k"
  Mux6/1 -> fcn3/1
  He_b/1 -> Mux6/1, BC1/3  "He_b"
  fcn3/1 -> BC1/4  "M0"
  Product1/1 -> pr_PHe/1
  Sum2/1 -> Product1/2
  HT/1 -> fcn1/1

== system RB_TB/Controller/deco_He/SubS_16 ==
  note: Model: RB_TB/Controller/deco_He/SubS_2
  Palv : Inport  Port=1  LatchInput=off
  Pamb_sea : Inport  Port=2  LatchInput=off
  Palv_INI : Inport  Port=3  LatchInput=off
  HT : Inport  Port=4  LatchInput=off
  BC1 : BusCreator  DialogController=Simulink.DDGSource_Bus
  He_a : Constant  Value=0.5109
  He_b : Constant  Value=0.9267
  Mux6 : Mux  Inputs=3
  Product1 : Product
  Sum2 : Sum  Inputs=|+-
  Sum3 : Sum  Inputs=++|
  fcn1 : Fcn  Expr=log(2)/u(1)
  fcn3 : Fcn  Expr=u(3)+u(2)/u(1)
  pr_PHe : TransferFcn  Numerator=[1/60]  Denominator=[1 0]
  bus : Outport
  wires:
  HT/1 -> fcn1/1
  Sum2/1 -> Product1/2
  Product1/1 -> pr_PHe/1
  fcn3/1 -> BC1/4  "M0"
  He_b/1 -> BC1/3, Mux6/1  "He_b"
  Mux6/1 -> fcn3/1
  fcn1/1 -> BC1/1, Product1/1  "He_k"
  Palv/1 -> Sum2/1
  Pamb_sea/1 -> Mux6/2
  He_a/1 -> Mux6/3  "He_a"
  Sum3/1 -> Sum2/2, BC1/2  "Pt"
  Palv_INI/1 -> Sum3/1
  pr_PHe/1 -> Sum3/2
  BC1/1 -> bus/1

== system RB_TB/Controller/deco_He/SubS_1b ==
  note: Model: RB_TB/Controller/deco_He/SubS_2
  Palv : Inport  Port=1  LatchInput=off
  Pamb_sea : Inport  Port=2  LatchInput=off
  Palv_INI : Inport  Port=3  LatchInput=off
  HT : Inport  Port=4  LatchInput=off
  BC1 : BusCreator  DialogController=Simulink.DDGSource_Bus
  He_a : Constant  Value=1.6236
  He_b : Constant  Value=0.4770
  Mux6 : Mux  Inputs=3
  Product1 : Product
  Sum2 : Sum  Inputs=|+-
  Sum3 : Sum  Inputs=++|
  fcn1 : Fcn  Expr=log(2)/u(1)
  fcn3 : Fcn  Expr=u(3)+u(2)/u(1)
  pr_PHe : TransferFcn  Numerator=[1/60]  Denominator=[1 0]
  bus : Outport
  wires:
  BC1/1 -> bus/1
  pr_PHe/1 -> Sum3/2
  Palv_INI/1 -> Sum3/1
  Sum3/1 -> BC1/2, Sum2/2  "Pt"
  He_a/1 -> Mux6/3  "He_a"
  Pamb_sea/1 -> Mux6/2
  Palv/1 -> Sum2/1
  fcn1/1 -> Product1/1, BC1/1  "He_k"
  Mux6/1 -> fcn3/1
  He_b/1 -> Mux6/1, BC1/3  "He_b"
  fcn3/1 -> BC1/4  "M0"
  Product1/1 -> pr_PHe/1
  Sum2/1 -> Product1/2
  HT/1 -> fcn1/1

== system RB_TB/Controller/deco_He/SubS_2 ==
  note: Model: RB_TB/Controller/deco_He/SubS_2
  Palv : Inport  Port=1  LatchInput=off
  Pamb_sea : Inport  Port=2  LatchInput=off
  Palv_INI : Inport  Port=3  LatchInput=off
  HT : Inport  Port=4  LatchInput=off
  BC1 : BusCreator  DialogController=Simulink.DDGSource_Bus
  He_a : Constant  Value=1.38
  He_b : Constant  Value=0.5747
  Mux6 : Mux  Inputs=3
  Product1 : Product
  Sum2 : Sum  Inputs=|+-
  Sum3 : Sum  Inputs=++|
  fcn1 : Fcn  Expr=log(2)/u(1)
  fcn3 : Fcn  Expr=u(3)+u(2)/u(1)
  pr_PHe : TransferFcn  Numerator=[1/60]  Denominator=[1 0]
  bus : Outport
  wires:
  HT/1 -> fcn1/1
  Sum2/1 -> Product1/2
  Product1/1 -> pr_PHe/1
  fcn3/1 -> BC1/4  "M0"
  He_b/1 -> BC1/3, Mux6/1  "He_b"
  Mux6/1 -> fcn3/1
  fcn1/1 -> BC1/1, Product1/1  "He_k"
  Palv/1 -> Sum2/1
  Pamb_sea/1 -> Mux6/2
  He_a/1 -> Mux6/3  "He_a"
  Sum3/1 -> Sum2/2, BC1/2  "Pt"
  Palv_INI/1 -> Sum3/1
  pr_PHe/1 -> Sum3/2
  BC1/1 -> bus/1

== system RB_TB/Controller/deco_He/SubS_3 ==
  note: Model: RB_TB/Controller/deco_He/SubS_2
  Palv : Inport  Port=1  LatchInput=off
  Pamb_sea : Inport  Port=2  LatchInput=off
  Palv_INI : Inport  Port=3  LatchInput=off
  HT : Inport  Port=4  LatchInput=off
  BC1 : BusCreator  DialogController=Simulink.DDGSource_Bus
  He_a : Constant  Value=1.1879
  He_b : Constant  Value=0.6527
  Mux6 : Mux  Inputs=3
  Product1 : Product
  Sum2 : Sum  Inputs=|+-
  Sum3 : Sum  Inputs=++|
  fcn1 : Fcn  Expr=log(2)/u(1)
  fcn3 : Fcn  Expr=u(3)+u(2)/u(1)
  pr_PHe : TransferFcn  Numerator=[1/60]  Denominator=[1 0]
  bus : Outport
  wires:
  BC1/1 -> bus/1
  pr_PHe/1 -> Sum3/2
  Palv_INI/1 -> Sum3/1
  Sum3/1 -> BC1/2, Sum2/2  "Pt"
  He_a/1 -> Mux6/3  "He_a"
  Pamb_sea/1 -> Mux6/2
  Palv/1 -> Sum2/1
  fcn1/1 -> Product1/1, BC1/1  "He_k"
  Mux6/1 -> fcn3/1
  He_b/1 -> Mux6/1, BC1/3  "He_b"
  fcn3/1 -> BC1/4  "M0"
  Product1/1 -> pr_PHe/1
  Sum2/1 -> Product1/2
  HT/1 -> fcn1/1

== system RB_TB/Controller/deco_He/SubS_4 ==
  note: Model: RB_TB/Controller/deco_He/SubS_2
  Palv : Inport  Port=1  LatchInput=off
  Pamb_sea : Inport  Port=2  LatchInput=off
  Palv_INI : Inport  Port=3  LatchInput=off
  HT : Inport  Port=4  LatchInput=off
  BC1 : BusCreator  DialogController=Simulink.DDGSource_Bus
  He_a : Constant  Value=1.0455
  He_b : Constant  Value=0.7223
  Mux6 : Mux  Inputs=3
  Product1 : Product
  Sum2 : Sum  Inputs=|+-
  Sum3 : Sum  Inputs=++|
  fcn1 : Fcn  Expr=log(2)/u(1)
  fcn3 : Fcn  Expr=u(3)+u(2)/u(1)
  pr_PHe : TransferFcn  Numerator=[1/60]  Denominator=[1 0]
  bus : Outport
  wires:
  HT/1 -> fcn1/1
  Sum2/1 -> Product1/2
  Product1/1 -> pr_PHe/1
  fcn3/1 -> BC1/4  "M0"
  He_b/1 -> BC1/3, Mux6/1  "He_b"
  Mux6/1 -> fcn3/1
  fcn1/1 -> BC1/1, Product1/1  "He_k"
  Palv/1 -> Sum2/1
  Pamb_sea/1 -> Mux6/2
  He_a/1 -> Mux6/3  "He_a"
  Sum3/1 -> Sum2/2, BC1/2  "Pt"
  Palv_INI/1 -> Sum3/1
  pr_PHe/1 -> Sum3/2
  BC1/1 -> bus/1

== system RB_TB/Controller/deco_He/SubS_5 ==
  note: Model: RB_TB/Controller/deco_He/SubS_2
  Palv : Inport  Port=1  LatchInput=off
  Pamb_sea : Inport  Port=2  LatchInput=off
  Palv_INI : Inport  Port=3  LatchInput=off
  HT : Inport  Port=4  LatchInput=off
  BC1 : BusCreator  DialogController=Simulink.DDGSource_Bus
  He_a : Constant  Value=0.9211
  He_b : Constant  Value=0.7582
  Mux6 : Mux  Inputs=3
  Product1 : Product
  Sum2 : Sum  Inputs=|+-
  Sum3 : Sum  Inputs=++|
  fcn1 : Fcn  Expr=log(2)/u(1)
  fcn3 : Fcn  Expr=u(3)+u(2)/u(1)
  pr_PHe : TransferFcn  Numerator=[1/60]  Denominator=[1 0]
  bus : Outport
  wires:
  BC1/1 -> bus/1
  pr_PHe/1 -> Sum3/2
  Palv_INI/1 -> Sum3/1
  Sum3/1 -> BC1/2, Sum2/2  "Pt"
  He_a/1 -> Mux6/3  "He_a"
  Pamb_sea/1 -> Mux6/2
  Palv/1 -> Sum2/1
  fcn1/1 -> Product1/1, BC1/1  "He_k"
  Mux6/1 -> fcn3/1
  He_b/1 -> Mux6/1, BC1/3  "He_b"
  fcn3/1 -> BC1/4  "M0"
  Product1/1 -> pr_PHe/1
  Sum2/1 -> Product1/2
  HT/1 -> fcn1/1

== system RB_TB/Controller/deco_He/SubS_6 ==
  note: Model: RB_TB/Controller/deco_He/SubS_2
  Palv : Inport  Port=1  LatchInput=off
  Pamb_sea : Inport  Port=2  LatchInput=off
  Palv_INI : Inport  Port=3  LatchInput=off
  HT : Inport  Port=4  LatchInput=off
  BC1 : BusCreator  DialogController=Simulink.DDGSource_Bus
  He_a : Constant  Value=0.8232
  He_b : Constant  Value=0.7957
  Mux6 : Mux  Inputs=3
  Product1 : Product
  Sum2 : Sum  Inputs=|+-
  Sum3 : Sum  Inputs=++|
  fcn1 : Fcn  Expr=log(2)/u(1)
  fcn3 : Fcn  Expr=u(3)+u(2)/u(1)
  pr_PHe : TransferFcn  Numerator=[1/60]  Denominator=[1 0]
  bus : Outport
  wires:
  HT/1 -> fcn1/1
  Sum2/1 -> Product1/2
  Product1/1 -> pr_PHe/1
  fcn3/1 -> BC1/4  "M0"
  He_b/1 -> BC1/3, Mux6/1  "He_b"
  Mux6/1 -> fcn3/1
  fcn1/1 -> BC1/1, Product1/1  "He_k"
  Palv/1 -> Sum2/1
  Pamb_sea/1 -> Mux6/2
  He_a/1 -> Mux6/3  "He_a"
  Sum3/1 -> Sum2/2, BC1/2  "Pt"
  Palv_INI/1 -> Sum3/1
  pr_PHe/1 -> Sum3/2
  BC1/1 -> bus/1

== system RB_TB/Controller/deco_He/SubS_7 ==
  note: Model: RB_TB/Controller/deco_He/SubS_2
  Palv : Inport  Port=1  LatchInput=off
  Pamb_sea : Inport  Port=2  LatchInput=off
  Palv_INI : Inport  Port=3  LatchInput=off
  HT : Inport  Port=4  LatchInput=off
  BC1 : BusCreator  DialogController=Simulink.DDGSource_Bus
  He_a : Constant  Value=0.7321
  He_b : Constant  Value=0.8279
  Mux6 : Mux  Inputs=3
  Product1 : Product
  Sum2 : Sum  Inputs=|+-
  Sum3 : Sum  Inputs=++|
  fcn1 : Fcn  Expr=log(2)/u(1)
  fcn3 : Fcn  Expr=u(3)+u(2)/u(1)
  pr_PHe : TransferFcn  Numerator=[1/60]  Denominator=[1 0]
  bus : Outport
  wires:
  BC1/1 -> bus/1
  pr_PHe/1 -> Sum3/2
  Palv_INI/1 -> Sum3/1
  Sum3/1 -> BC1/2, Sum2/2  "Pt"
  He_a/1 -> Mux6/3  "He_a"
  Pamb_sea/1 -> Mux6/2
  Palv/1 -> Sum2/1
  fcn1/1 -> Product1/1, BC1/1  "He_k"
  Mux6/1 -> fcn3/1
  He_b/1 -> Mux6/1, BC1/3  "He_b"
  fcn3/1 -> BC1/4  "M0"
  Product1/1 -> pr_PHe/1
  Sum2/1 -> Product1/2
  HT/1 -> fcn1/1
